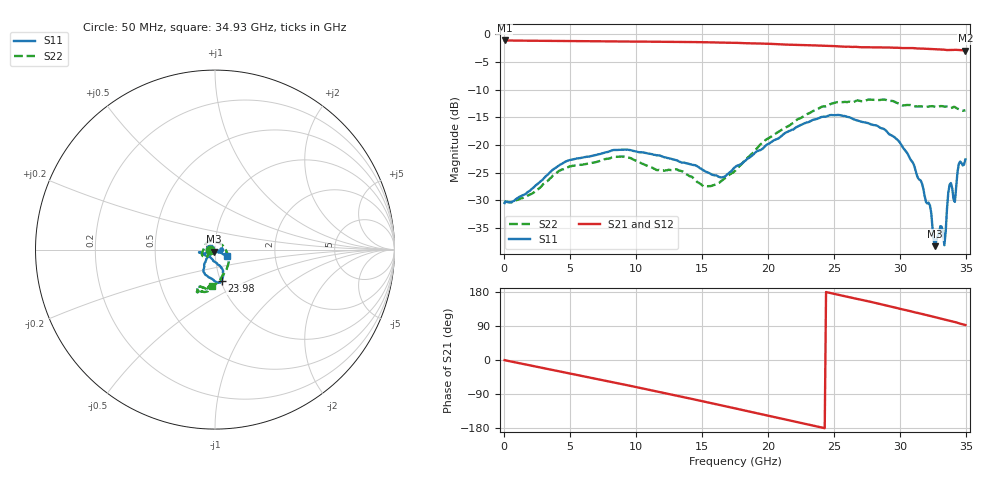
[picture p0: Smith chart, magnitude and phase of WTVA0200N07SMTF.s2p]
! 50 ohm 2-Port S-parameters measured by Modelithics Inc support@modelithics.com  Tampa, FL USA 813-866-6335 (February 2024)
! Smiths Interconnect,  2dB P/N: WTVA0200N07SMTF, Temperature: 125 C
! Board: 10 mil Rogers 4350B, Mounting Pad Dimensions: Length: 15 mils, Width: 25 mils, Gap: 40 mils.
# Hz S RI R 50
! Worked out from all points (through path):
!   352 points, 50 MHz to 34.93 GHz, reference 50 ohm
!   highest |S21| = -1.11 dB at 50 MHz (marker M1); lowest = -3.0 dB at 34.93 GHz (marker M2)
!   group delay of S21, straight-line fit = 21.1 ps
!   lowest |S11| = -38.3 dB at 32.64 GHz (marker M3), VSWR 1.02, Z = 49.4 - j1.05 ohm
!   |S11| at or under -10 dB: start of sweep to end of sweep
!   |S22| runs from -30.5 to -11.8 dB; largest |S21 - S12| = 0.009
!   S11 on the Smith chart (normalised r, x): 50 MHz: 0.94, +0.00; 23.98 GHz: 1.01, -0.36; 34.93 GHz: 1.14, -0.08
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5e7  -0.0298 0.000988  0.8798 -0.00525  0.8785 -0.00505  -0.0298 2.33e-05
5.8715e9  -0.0735 -0.021  0.6455 -0.5783  0.6446 -0.5775  -0.0494 -0.0437
9.0555e9  -0.0891 -0.0148  0.37 -0.777  0.3684 -0.7762  -0.073 -0.0285
1.1742e10  -0.078 -0.019  0.0882 -0.8516  0.0866 -0.8505  -0.0566 0.0181
1.5125e10  -0.0479 -0.0339  -0.2838 -0.7991  -0.2855 -0.7973  0.00522 0.0417
1.6518e10  -0.0251 -0.0441  -0.4225 -0.7276  -0.4231 -0.7259  0.0409 0.0247
1.7513e10  -0.00949 -0.0625  -0.5134 -0.6617  -0.5128 -0.6604  0.0584 0.000478
1.98015e10  0.0303 -0.0936  -0.6781 -0.4655  -0.677 -0.4649  0.0735 -0.0826
2.33835e10  0.0411 -0.1632  -0.7875 -0.098  -0.7862 -0.0986  -0.00717 -0.202
2.39805e10  0.0364 -0.174  -0.7888 -0.0318  -0.7875 -0.0334  -0.0236 -0.2176
2.91545e10  -0.0628 -0.108  -0.6001 0.4658  -0.5948 0.47  -0.0977 -0.2296
3.0448e10  -0.0531 -0.0686  -0.4992 0.5615  -0.4935 0.5649  -0.0845 -0.2137
3.1642e10  -0.0308 -0.0323  -0.3881 0.6336  -0.3849 0.634  -0.0813 -0.207
3.19405e10  -0.0206 -0.0224  -0.3569 0.6482  -0.3548 0.6478  -0.0734 -0.208
3.2239e10  -0.0178 -0.0222  -0.3269 0.6593  -0.3233 0.6594  -0.071 -0.2115
3.2637e10  -0.00589 -0.0106  -0.2871 0.6745  -0.2836 0.6744  -0.0635 -0.2115
3.3035e10  0.0138 -0.0121  -0.2437 0.687  -0.238 0.6876  -0.0546 -0.2176
3.33335e10  0.0119 -0.00348  -0.2109 0.6946  -0.2073 0.6944  -0.0559 -0.2146
3.37315e10  0.0424 -0.00998  -0.1697 0.7015  -0.1645 0.7014  -0.0456 -0.2129
3.41295e10  0.0296 -0.00743  -0.1321 0.7123  -0.1259 0.7121  -0.0426 -0.2161
3.4428e10  0.0614 -0.0271  -0.0869 0.7156  -0.0857 0.7144  -0.0317 -0.2083
3.49255e10  0.0663 -0.0329  -0.0291 0.7105  -0.0291 0.7089  -0.0177 -0.2046
